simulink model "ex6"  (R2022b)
settings: Solver=ode45  StartTime=0.0  StopTime=10.0  RelTol=1e-3  EnableMultiTasking=on

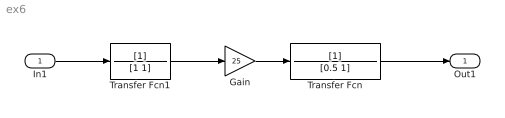
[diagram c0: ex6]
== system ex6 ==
  In1 : Inport
  Gain : Gain  Gain=25
  Transfer Fcn : TransferFcn  Denominator=[0.5 1]
  Transfer Fcn1 : TransferFcn  Denominator=[1 1]
  Out1 : Outport
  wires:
  Transfer Fcn1/1 -> Gain/1
  Gain/1 -> Transfer Fcn/1
  In1/1 -> Transfer Fcn1/1
  Transfer Fcn/1 -> Out1/1
